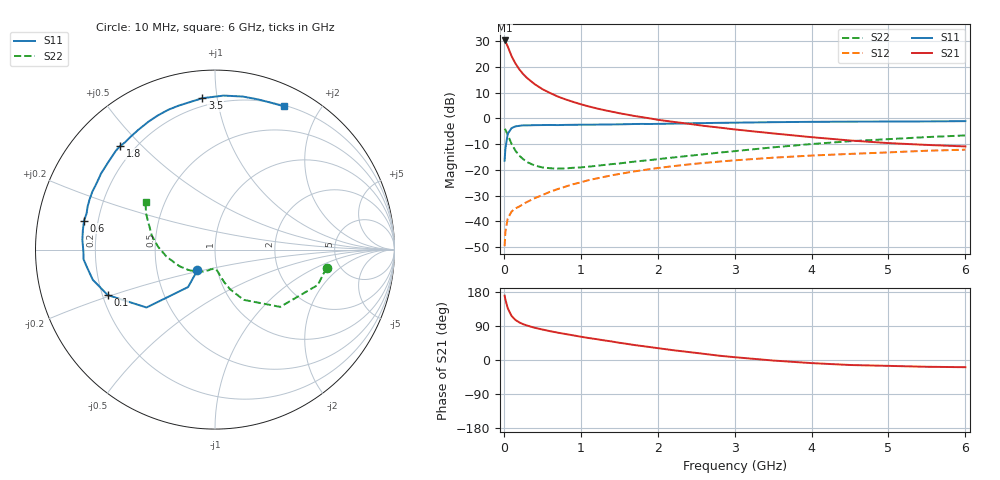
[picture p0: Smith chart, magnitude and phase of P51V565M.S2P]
! SIEMENS Small Signal Semiconductors
! BFP183
! Si NPN RF Bipolar Junction Transistor in SOT143
! VCE = 1.5 V  IC = 65 mA
! Common Emitter S-Parameters:  March  1996
# GHz  S  MA  R  50
!  f  S11  S21  S12  S22
! GHz  MAG  ANG  MAG  ANG  MAG  ANG  MAG  ANG
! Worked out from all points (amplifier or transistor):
!   36 points, 10 MHz to 6 GHz, reference 50 ohm
!   highest |S21| = 30.3 dB at 10 MHz (marker M1)
!   |S21| within 3 dB of that: start of sweep to 59.23 MHz
!   unconditionally stable (mu >= 1): start of sweep to 43.08 MHz; 115.7 MHz to end of sweep
!   at 250 MHz: K = 1.40, MAG = 21.5 dB, |S12| = -33.3 dB
!   at 1.4 GHz: K = 1.94, MAG = 6.8 dB, |S12| = -22.1 dB
!   at 6 GHz: K = 1.54, MAG = -3.7 dB, |S12| = -12.1 dB
!   S11 on the Smith chart (normalised r, x): 10 MHz: 0.80, -0.19; 100 MHz: 0.22, -0.19; 600 MHz: 0.15, +0.11; 1.8 GHz: 0.15, +0.43; 3.5 GHz: 0.15, +0.91; 6 GHz: 0.21, +1.57
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0.01  0.1514 -130.4  32.75 169.9  0.0033 57.1  0.6296 -9.3
0.02  0.2571 -125.7  31.49 160.2  0.0062 61.4  0.6057 -19.0
0.05  0.4997 -139.8  25.11 136.9  0.0113 54.0  0.4835 -41.3
0.1  0.6491 -157.0  16.32 116.4  0.0155 42.7  0.3222 -60.3
0.15  0.7012 -166.1  11.72 105.8  0.0179 43.3  0.2373 -69.1
0.2  0.7187 -171.8  9.041 99.3  0.0194 45.1  0.1898 -74.1
0.25  0.7344 -175.8  7.32 94.6  0.0216 47.3  0.1624 -77.0
0.3  0.7334 -179.3  6.141 91.1  0.0238 49.9  0.1427 -79.5
0.4  0.741 175.8  4.644 85.1  0.0282 55.1  0.1218 -83.2
0.5  0.7441 171.6  3.719 80.5  0.0324 57.4  0.112 -86.5
0.6  0.7472 167.5  3.131 76.1  0.0376 58.7  0.1077 -89.3
0.7  0.7431 164.3  2.669 72.2  0.0424 60.2  0.1062 -92.3
0.8  0.7492 161.4  2.351 68.6  0.0473 60.6  0.1069 -95.0
1.1  0.7554 151.9  1.718 58.1  0.0632 60.9  0.1155 -104.1
1.5  0.7683 141.0  1.265 45.5  0.0834 58.4  0.1335 -115.8
1.8  0.7826 132.5  1.058 36.8  0.0986 55.8  0.1503 -125.3
2.2  0.7925 122.6  0.86 25.9  0.1184 51.4  0.1742 -137.5
2.8  0.8215 108.4  0.665 11.3  0.1452 44.2  0.2168 -154.4
3.5  0.8465 94.8  0.512 -1.4  0.1728 36.3  0.2746 -172.2
4.5  0.8667 79.7  0.373 -13.2  0.2047 24.8  0.361 167.3
5.5  0.876 69.0  0.306 -17.9  0.236 14.9  0.4345 152.2
6  0.8862 64.3  0.286 -19.0  0.2473 9.5  0.4678 145.8
